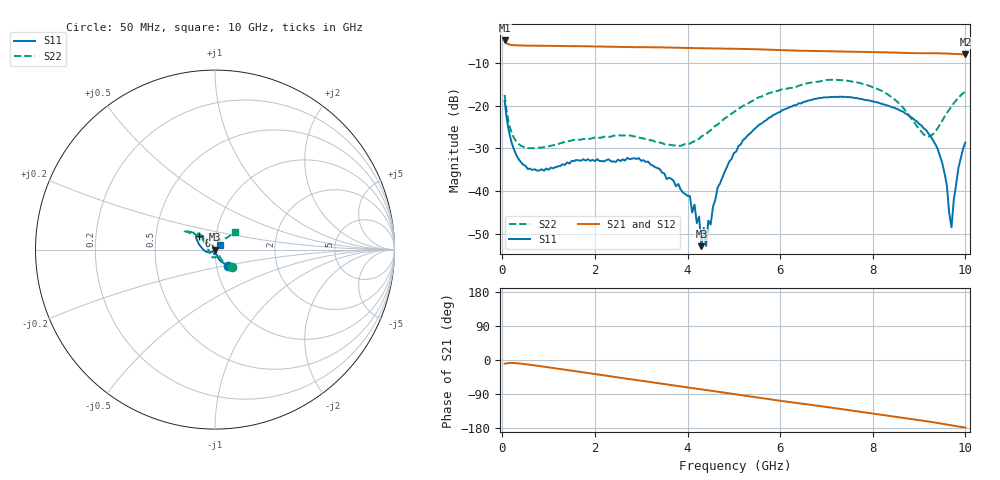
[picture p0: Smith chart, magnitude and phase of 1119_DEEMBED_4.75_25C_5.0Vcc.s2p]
!Hittite Microwave Corp.
!Digital Attenuator/PhaseShifter Rev 1.4.0
!Filename: C:\DATA\DATA\1119_DEEMBED_4.75_25C_5.0Vcc.s2p
!VNA ID: Agilent Technologies,N5224A,MY51441122,A.10.45.03
!Device type:
!2 Port Calibration.
!Temp(C): 25
!Lot Number:
!Serial Number:
!Operator:
!Misc:
!Attenuator:  4.750
# GHZ S DB R 50.0
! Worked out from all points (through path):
!   200 points, 50 MHz to 10 GHz, reference 50 ohm
!   highest |S21| = -4.75 dB at 50 MHz (marker M1); lowest = -8.0 dB at 10 GHz (marker M2)
!   group delay of S21, straight-line fit = 48.3 ps
!   lowest |S11| = -52.9 dB at 4.3 GHz (marker M3), VSWR 1.00, Z = 50.2 - j0.0983 ohm
!   |S11| at or under -10 dB: start of sweep to end of sweep
!   |S22| runs from -30.0 to -13.9 dB; largest |S21 - S12| = 0.0017
!   S11 on the Smith chart (normalised r, x): 50 MHz: 1.13, -0.21; 6.7 GHz: 0.83, +0.13; 10 GHz: 1.05, +0.06
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0.05  -18.86 -52.2  -4.75 -9.9  -4.75 -9.9  -17.49 -46.2
0.2  -28.61 -71.8  -5.81 -7.7  -5.81 -7.7  -26.29 -56.7
0.55  -34.81 -73.3  -5.96 -11.8  -5.96 -11.8  -29.90 -52.1
1.75  -32.53 -98.8  -6.10 -32.6  -6.11 -32.7  -27.80 -80.0
3.4  -34.82 -88.2  -6.36 -61.7  -6.37 -61.7  -28.61 -136.4
4.05  -41.10 -60.7  -6.50 -73.2  -6.51 -73.3  -28.86 -175.9
4.25  -45.92 -25.4  -6.56 -76.8  -6.57 -76.8  -27.74 170.5
4.3  -52.85 -25.4  -6.57 -77.6  -6.59 -77.7  -27.18 166.3
4.35  -48.56 20.5  -6.58 -78.4  -6.59 -78.5  -26.94 162.5
4.4  -52.82 28.1  -6.58 -79.4  -6.60 -79.5  -26.65 160.7
4.45  -46.87 69.7  -6.60 -80.3  -6.62 -80.3  -26.10 158.2
4.5  -47.80 75.8  -6.61 -81.0  -6.63 -81.1  -25.78 155.5
4.65  -39.11 104.5  -6.63 -83.7  -6.65 -83.7  -24.41 149.0
5.05  -30.72 121.9  -6.70 -90.7  -6.72 -90.7  -21.11 140.7
6.7  -18.56 139.0  -7.20 -119.0  -7.21 -119.0  -14.51 147.6
8.35  -20.07 158.7  -7.55 -147.7  -7.56 -147.7  -17.55 137.3
9.1  -25.29 -171.4  -7.73 -160.5  -7.74 -160.5  -26.70 112.6
9.35  -29.00 -154.7  -7.74 -165.2  -7.76 -165.2  -26.07 73.3
9.55  -35.83 -135.3  -7.79 -169.2  -7.81 -169.2  -22.57 51.0
9.7  -48.46 -59.1  -7.86 -172.3  -7.88 -172.3  -20.17 44.4
9.85  -34.53 39.6  -7.94 -175.3  -7.95 -175.3  -18.14 42.5
10  -28.62 47.1  -8.03 -178.4  -8.04 -178.4  -16.67 41.5
